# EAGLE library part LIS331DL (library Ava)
MEMS motion sensor
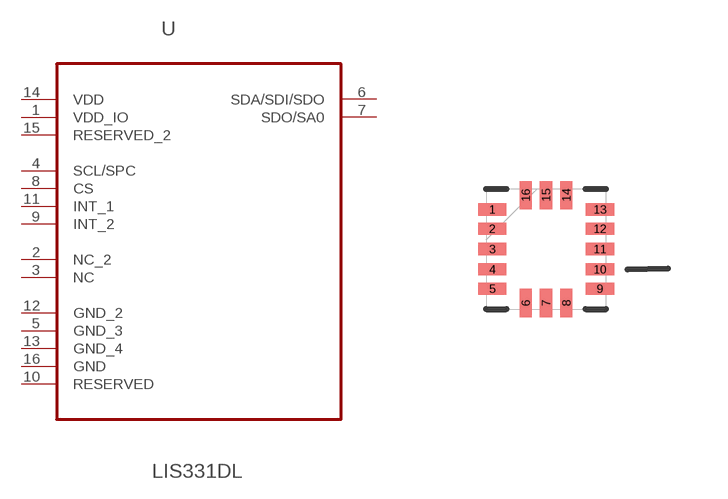
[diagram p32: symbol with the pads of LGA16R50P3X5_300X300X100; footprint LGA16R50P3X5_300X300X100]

Designator prefix U

## LIS331DL (MPN: LIS331DL; OC_FARNELL: 1838521; OC_NEWARK: 56P7989; PACKAGE: LGA-16; SUPPLIER: STMicroelectronics)  [LGA16R50P3X5_300X300X100]
1  VDD_IO  pwr
2  NC_2  nc
3  NC  nc
4  SCL/SPC  in
5  GND_3  pas
6  SDA/SDI/SDO
7  SDO/SA0  out
8  CS  in
9  INT_2  in
10  RESERVED  pas
11  INT_1  in
12  GND_2  pas
13  GND_4  pas
14  VDD  pwr
15  RESERVED_2  pwr
16  GND  pas

## Footprint LGA16R50P3X5_300X300X100 (pad centres in mm)
smd 0.711 x 0.305: 1 -1.346,0.991; 2 -1.346,0.508; 3 -1.346,0; 4 -1.346,-0.508; 5 -1.346,-0.991; 9 1.346,-0.991; 10 1.346,-0.508; 11 1.346,0; 12 1.346,0.508; 13 1.346,0.991
smd 0.305 x 0.711: 6 -0.508,-1.346; 7 0,-1.346; 8 0.508,-1.346; 14 0.508,1.346; 15 0,1.346; 16 -0.508,1.346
